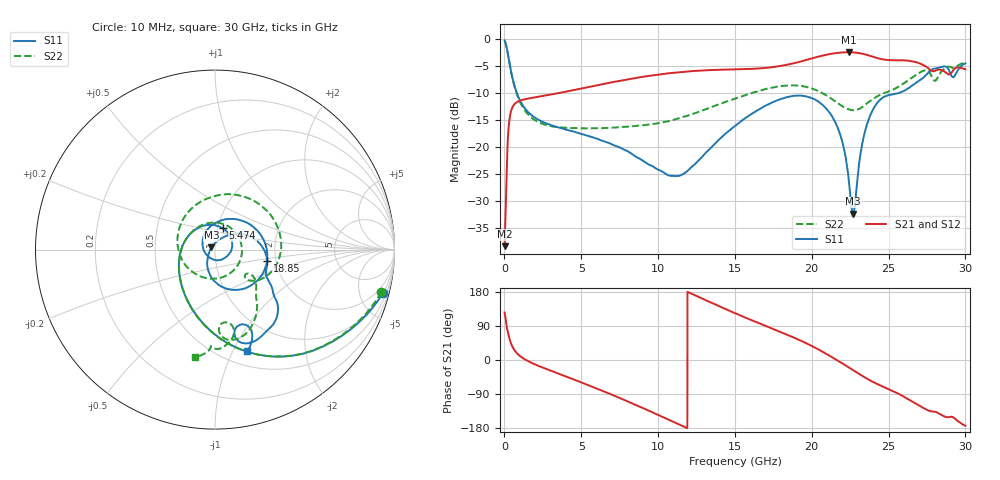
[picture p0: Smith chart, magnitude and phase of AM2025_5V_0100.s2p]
!Keysight Technologies,N5245B,MY58422270,A.16.20.02
!Date: Tuesday, July 14, 2026 01:03:47
!Correction: S11(C  2-Port  )
!S21(C  2-Port  )
!S12(C  2-Port  )
!S22(C  2-Port  )
!S2P File: Measurements: S11, S21, S12, S22:
# Hz S  dB  R 50
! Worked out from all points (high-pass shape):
!   3201 points, 10 MHz to 30 GHz, reference 50 ohm
!   highest |S21| = -2.48 dB at 22.42 GHz (marker M1); lowest = -38.3 dB at 10 MHz (marker M2)
!   |S21| within 3 dB of the highest: 16.5 GHz to 27.61 GHz (11.11 GHz wide, 50.4 % of centre); 29.31 GHz to 29.83 GHz (520.9 MHz wide, 1.76 % of centre)
!   lowest |S11| = -32.3 dB at 22.69 GHz (marker M3), VSWR 1.05, Z = 48 + j1.23 ohm
!   |S11| at or under -10 dB: 804.4 MHz to 25.69 GHz (24.89 GHz wide, 188 % of centre)
!   |S22| runs from -16.5 to -0.4 dB; largest |S21 - S12| = 0.012
!   S11 on the Smith chart (normalised r, x): 10 MHz: 1.07, -7.70; 5.474 GHz: 1.06, +0.26; 18.85 GHz: 1.79, -0.26; 30 GHz: 0.65, -1.14
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1e7  -0.30 -14.5  -38.31 125.2  -37.30 170.9  -0.39 -14.3
3.005281e8  -4.07 -68.6  -15.50 60.4  -15.51 60.3  -4.12 -69.2
5.816844e8  -7.94 -101.9  -12.34 30.5  -12.36 30.5  -8.06 -103.2
2.212391e9  -14.96 169.1  -10.70 -15.5  -10.70 -15.5  -15.39 158.3
5.014581e9  -17.57 82.3  -9.18 -59.2  -9.18 -59.3  -16.53 54.3
5.473803e9  -17.95 69.6  -8.91 -66.5  -8.91 -66.6  -16.54 39.3
7.873003e9  -20.60 2.6  -7.57 -106.7  -7.57 -106.8  -16.26 -37.8
1.000979e10  -24.21 -73.8  -6.61 -144.9  -6.61 -144.9  -15.58 -107.6
1.161238e10  -25.03 -155.5  -6.10 -174.5  -6.10 -174.6  -14.45 -158.2
1.5005e10  -16.11 83.8  -5.65 123.5  -5.65 123.5  -11.05 105.3
1.688875e10  -12.50 37.5  -5.40 91.8  -5.40 91.7  -9.36 57.9
1.884747e10  -10.53 -12.7  -4.51 59.0  -4.50 59.0  -8.60 9.8
2.000958e10  -10.98 -45.2  -3.62 36.8  -3.61 36.8  -9.16 -16.5
2.16028e10  -15.84 -95.8  -2.63 0.6  -2.62 0.6  -11.71 -41.8
2.241815e10  -26.25 -140.1  -2.48 -19.8  -2.48 -19.8  -13.04 -42.1
2.268994e10  -32.32 148.0  -2.51 -26.7  -2.51 -26.8  -13.21 -40.0
2.359901e10  -15.78 32.7  -2.98 -49.4  -2.97 -49.4  -11.91 -34.7
2.500479e10  -10.41 -16.2  -3.93 -76.8  -3.93 -76.9  -9.71 -45.6
2.717907e10  -7.39 -38.7  -4.74 -124.7  -4.74 -124.9  -6.01 -70.5
2.803191e10  -5.48 -54.6  -5.91 -136.4  -5.92 -136.5  -7.76 -81.8
2.899721e10  -6.24 -77.1  -6.55 -150.1  -6.54 -150.3  -5.19 -90.8
3e10  -4.54 -72.5  -5.62 -173.5  -5.61 -173.6  -4.30 -100.4
